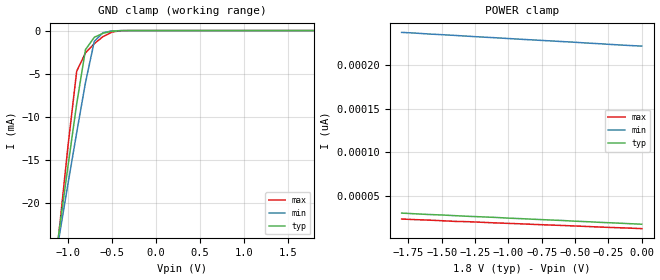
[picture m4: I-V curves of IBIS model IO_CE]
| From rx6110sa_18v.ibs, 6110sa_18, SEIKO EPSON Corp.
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[Model]   IO_CE
Model_type Input
Enable Active-High
Polarity Non-Inverting
Vinh=1.26
Vinl=0.54
C_comp   2.5p   2p   3p
[Temperature Range] 25   85   -40
[Voltage Range]   1.8   1.6   2.0
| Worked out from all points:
|   GND clamp passes 1 mA (typ) near -0.72 V on its own axis
[GND Clamp]
-1.8V     -77.83mA   -68.37mA   -94.23mA
-1.1V     -23.27mA   -23.92mA   -23.27mA
-1V       -15.78mA   -17.8mA    -13.47mA
-900mV    -8.484mA   -11.82mA   -4.704mA
-800mV    -2.203mA   -6.011mA   -2.581mA
-700mV    -778.2uA   -1.248mA   -1.513mA
-600mV    -308.4uA   -237.7uA   -691.7uA
-500mV    -74.64uA   -42.19uA   -176.5uA
-400mV    -7.865uA   -4.915uA   -14.75uA
1.8V      17.28pA    223.9pA    11.03pA
[POWER Clamp]
-1.8V     30.13pA    238.1pA    23.31pA
-1.7V     29.33pA    237.3pA    22.62pA
-1.6V     28.54pA    236.2pA    22.06pA
-1.5V     27.97pA    235.4pA    21.37pA
-1.4V     27.17pA    234.6pA    20.58pA
-1.3V     26.43pA    233.6pA    20.24pA
-1.1V     25.18pA    231.9pA    18.87pA
-1V       24.33pA    231pA      18.3pA
-600mV    21.66pA    227.5pA    15.92pA
-500mV    20.8pA     226.7pA    15.29pA
-200mV    18.76pA    223.9pA    13.42pA
0V        17.34pA    222.3pA    12.22pA
